(* Logix 5000 DataType export VMP_Cfg; software revision 30.00 *)

TYPE VMP_Cfg :
STRUCT
   ReadyInterlock : BOOL;   // RdyInputEnabled
   CEthernetRunReady : BOOL;   // EthSendBusy
   HoldOnFault : BOOL;   // HoldOnFault
   Spare1_3 : BOOL;   // Spare Bit
   Spare1_4 : BOOL;   // Spare Bit
   Spare1_5 : BOOL;   // Spare Bit
   Spare1_6 : BOOL;   // Spare Bit
   Spare1_7 : BOOL;   // Spare Bit
   SpareByte1 : SINT; {access Read Only}   // Spare data1
   SpareByte2 : SINT; {access Read Only}   // Spare data1
END_STRUCT
END_TYPE
